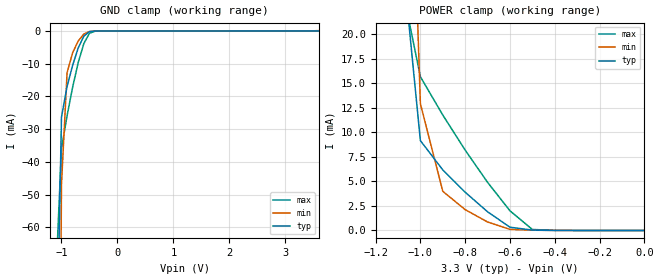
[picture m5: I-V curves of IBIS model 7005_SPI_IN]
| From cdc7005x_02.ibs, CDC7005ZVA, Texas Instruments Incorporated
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| Device Control Input Receiver Model SPI LOGIC
[Model]   7005_SPI_IN
Model_type  Input
Polarity   Non-Inverting
Vinl = 0.8V
Vinh = 2.0V
| variable   typ   min   max
C_comp   0.57p   NA   NA
[Temperature Range]   27   125   -20
[Voltage range]   3.3   3.0   3.6
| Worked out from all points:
|   GND clamp passes 1 mA (typ) near -0.56 V on its own axis
|   POWER clamp passes 1 mA (typ) near -0.64 V on its own axis
|Process range|   nominal   weak   strong
[POWER Clamp]
|   27C:3.3V:nominal   125C:3.0V:weak   -20C:3.6V:strong
|  Voltage   I(typ)   I(min)   I(max)
-3.6V     4.178A     3.281A     5.394A
-1.1V     32.37mA    81.73mA    26.86mA
-1V       9.161mA    12.93mA    15.68mA
-900mV    6.177mA    3.995mA    11.77mA
-800mV    3.901mA    2.123mA    8.192mA
-700mV    1.906mA    865.1uA    4.907mA
-600mV    331.8uA    112.7uA    2.004mA
-500mV    36.71uA    28.06uA    101.9uA
-400mV    5.784uA    5.867uA    13.59uA
0V        79.56pA    1.099nA    66.3pA
[GND Clamp]
|   27C:3.3V:nominal   125C:3.0V:weak   -20C:3.6V:strong
|  Voltage   I(typ)   I(min)   I(max)
-3.6V     -12.56A    -9.883A    -16.21A
-1.1V     -114.2mA   -281.5mA   -75.2mA
-1V       -26.33mA   -46.87mA   -35.96mA
-900mV    -16.97mA   -12.73mA   -25.9mA
-800mV    -10.45mA   -6.621mA   -17.11mA
-700mV    -5.142mA   -3.063mA   -9.584mA
-600mV    -1.579mA   -944.1uA   -3.825mA
-500mV    -228.8uA   -183.3uA   -720.8uA
-400mV    -38.27uA   -40.02uA   -72.69uA
3.6V      2.152uA    112.7uA    66.3pA
